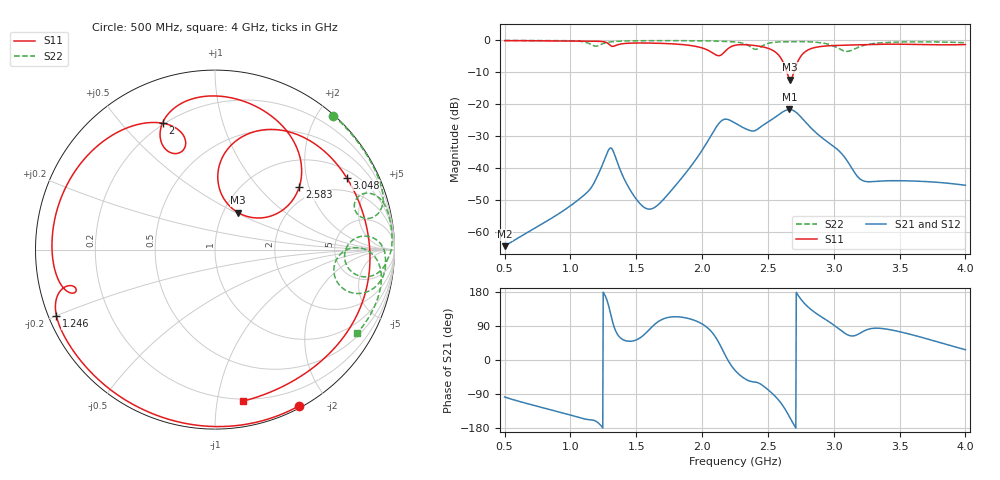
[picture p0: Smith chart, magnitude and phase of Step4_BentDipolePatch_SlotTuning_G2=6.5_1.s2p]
! TOUCHSTONE file generated by CST MICROWAVE STUDIO
! Date and time: Wed May 20 00:46:37 2020
! Project name: DualBand_DualMode_Antenna_FD_SteppedDesign.cst
! Parameters = {FPL=20; FPW=20; L=50; ST=10; SW=30; W=52; WF=7; ext=10; gap=1; inset=13}
! Header version: 2015
! Port assignment regex: !\s*Touchstone port\s*([0-9]+)\s*=\s*CST MWS port\s*([0-9]+)\s*\(\"(.*)\"\)(\s*mode\s*([0-9]+))?.*
! Touchstone port assignment:
! Touchstone port 1 = CST MWS port 1 ("")
! Touchstone port 2 = CST MWS port 2 ("")
# GHz S MA R 50
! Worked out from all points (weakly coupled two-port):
!   1006 points, 500 MHz to 4 GHz, reference 50 ohm
!   highest |S21| = -21.68 dB at 2.663 GHz (marker M1); lowest = -64.6 dB at 500 MHz (marker M2)
!   lowest |S11| = -12.3 dB at 2.67 GHz (marker M3), VSWR 1.64, Z = 58.8 + j25.7 ohm
!   |S11| at or under -10 dB: 2.644 GHz to 2.697 GHz (52.79 MHz wide, 1.98 % of centre)
!   |S22| runs from -3.5 to 0.0 dB; largest |S21 - S12| = 3.4e-05
!   S11 on the Smith chart (normalised r, x): 500 MHz: 0.02, -1.67; 1.246 GHz: 0.02, -0.20; 2 GHz: 0.20, +0.65; 2.583 GHz: 1.63, +1.73; 3.048 GHz: 1.30, +3.46; 4 GHz: 0.18, -1.19
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0.5  0.9886 -61.8  0.000592 -97.6  0.000592 -97.6  0.9966 48.6
0.787  0.9833 -97.2  0.00133 -125.6  0.001329 -125.6  0.996 28.8
1.0845  0.9722 -134.2  0.003467 -153.5  0.003464 -153.7  0.9601 14.4
1.2455  0.9577 -157.2  0.01148 -179.2  0.01149 -179.2  0.8852 20.6
1.312  0.8116 -165.3  0.02021 112.2  0.0202 112.2  0.9491 18.3
1.5185  0.9094 175.9  0.002899 56.2  0.002899 56.3  0.9863 11.7
1.669  0.9004 156.6  0.002674 101.8  0.002675 101.8  0.9897 8.2
2  0.7609 112.4  0.01888 95.2  0.01888 95.2  0.9849 1.1
2.1415  0.5854 113.6  0.05347 36.5  0.05348 36.5  0.9683 -2.4
2.25  0.8367 102.8  0.0504 -27.2  0.0504 -27.2  0.9452 -5.9
2.404  0.8275 73.3  0.03856 -58.3  0.03856 -58.3  0.7232 -3.3
2.46  0.7917 63.0  0.04631 -67.2  0.04632 -67.2  0.8275 5.2
2.5825  0.5843 36.6  0.06836 -106.3  0.06837 -106.3  0.9442 -0.6
2.663  0.2509 49.0  0.08243 -149.2  0.08243 -149.2  0.9518 -3.6
2.67  0.2431 57.7  0.08231 -153.7  0.0823 -153.7  0.9521 -3.8
2.7295  0.4766 86.9  0.06962 170.7  0.06962 170.7  0.9545 -5.7
2.8345  0.7503 63.0  0.04091 131.2  0.04091 131.2  0.944 -9.9
3.048  0.8358 28.7  0.0178 79.8  0.0178 79.8  0.7245 -16.1
3.2125  0.8539 8.6  0.006443 73.3  0.006447 73.4  0.8151 0.6
3.419  0.8715 -15.8  0.006289 80.5  0.006289 80.5  0.9305 -7.1
3.6955  0.8571 -47.2  0.006108 57.1  0.006108 57.1  0.9463 -16.8
4  0.8585 -79.4  0.005337 27.2  0.005337 27.2  0.919 -30.4
